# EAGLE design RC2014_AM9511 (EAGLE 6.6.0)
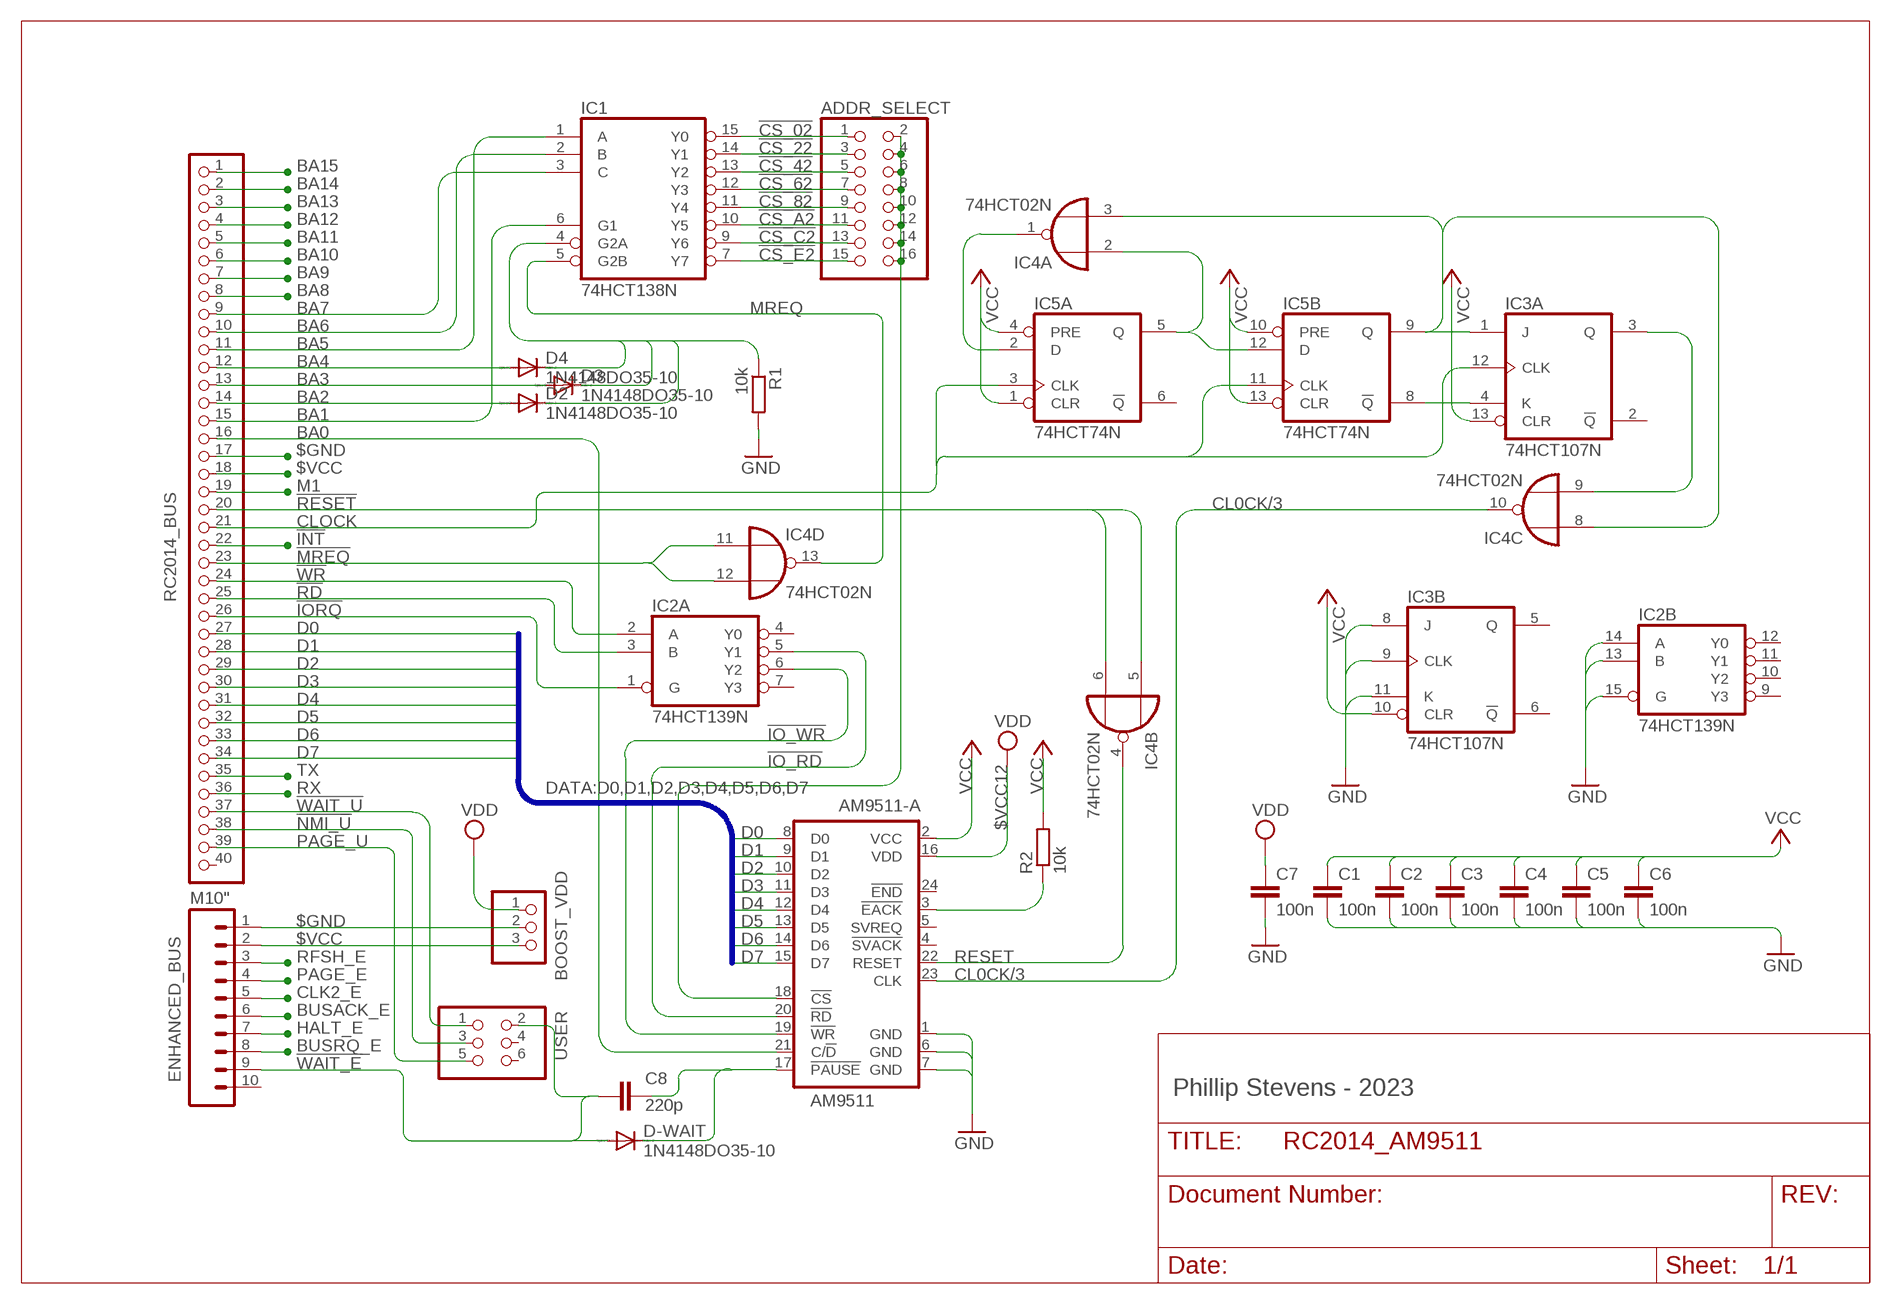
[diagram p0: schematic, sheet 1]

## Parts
ADDR_SELECT  PINHD-2X8  [2X08]
AM9511-A  AM9511  [DIL24-6]
BOOST_VDD  PINHD-1X3  [1X03]
C1  100n  C-EU025-025X050  [C025-025X050]
C2  100n  C-EU025-025X050  [C025-025X050]
C3  100n  C-EU025-025X050  [C025-025X050]
C4  100n  C-EU025-025X050  [C025-025X050]
C5  100n  C-EU025-025X050  [C025-025X050]
C6  100n  C-EU025-025X050  [C025-025X050]
C7  100n  C-EU025-025X050  [C025-025X050]
C8  220p  C-EU025-025X050  [C025-025X050]
D2  1N4148DO35-10  [DO35-10]
D3  1N4148DO35-10  [DO35-10]
D4  1N4148DO35-10  [DO35-10]
D-WAIT  1N4148DO35-10  [DO35-10]
ENHANCED_BUS  M10"  [1X10]
IC1  74HCT138N  [DIL16]
IC2  74HCT139N  [DIL16]
IC3  74HCT107N  [DIL14]
IC4  74HCT02N  [DIL14]
IC5  74HCT74N  [DIL14]
R1  10k  R-EU_0207/10  [0207/10]
R2  10k  R-EU_0207/10  [0207/10]
RC2014_BUS  RC2014 BUS  PINHD-1X40  [1X40]
USER  PINHD-2X3  [2X03]

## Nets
!CS: ADDR_SELECT.2 ADDR_SELECT.4 ADDR_SELECT.6 ADDR_SELECT.8 ADDR_SELECT.10 ADDR_SELECT.12 ADDR_SELECT.14 ADDR_SELECT.16 AM9511-A.18(!CS)
!CS_02: ADDR_SELECT.1 IC1.15(Y0)
!CS_22: ADDR_SELECT.3 IC1.14(Y1)
!CS_42: ADDR_SELECT.5 IC1.13(Y2)
!CS_62: ADDR_SELECT.7 IC1.12(Y3)
!CS_82: ADDR_SELECT.9 IC1.11(Y4)
!CS_A2: ADDR_SELECT.11 IC1.10(Y5)
!CS_C2: ADDR_SELECT.13 IC1.9(Y6)
!CS_E2: ADDR_SELECT.15 IC1.7(Y7)
!EACK: AM9511-A.3(!EACK) R2.1
!INT: RC2014_BUS.22
!IO_RD: AM9511-A.20(!RD) IC2.5(A:Y1)
!IO_WR: AM9511-A.19(!WR) IC2.6(A:Y2)
!IORQ: IC2.1(A:G) RC2014_BUS.26
!MREQ: IC4.11(D:I0) IC4.12(D:I1) RC2014_BUS.23
!NMI_U: RC2014_BUS.38 USER.3
!PAUSE: AM9511-A.17(!PAUSE) C8.1 D-WAIT.C
!RD: IC2.3(A:B) RC2014_BUS.25
!RESET: IC4.5(B:I0) IC4.6(B:I1) RC2014_BUS.20
!WAIT_E: C8.2 D-WAIT.A ENHANCED_BUS.9 USER.2
!WAIT_U: RC2014_BUS.37 USER.1
!WR: IC2.2(A:A) RC2014_BUS.24
$GND: AM9511-A.1(GND) AM9511-A.6(GND) AM9511-A.7(GND) BOOST_VDD.2 C1.2 C2.2 C3.2 C4.2 C5.2 C6.2 C7.2 ENHANCED_BUS.1 IC2.13(B:B) IC2.14(B:A) IC2.15(B:G) IC3.8(B:J) IC3.9(B:CLK) IC3.11(B:K) R1.2 RC2014_BUS.17 ; supply symbol labelled GND
$VCC: AM9511-A.2(VCC) BOOST_VDD.3 C1.1 C2.1 C3.1 C4.1 C5.1 C6.1 ENHANCED_BUS.2 IC3.10(B:CLR) IC3.13(A:CLR) IC5.1(A:CLR) IC5.4(A:PRE) IC5.10(B:PRE) IC5.13(B:CLR) R2.2 RC2014_BUS.18 ; supply symbol labelled VCC
$VCC12: AM9511-A.16(VDD) BOOST_VDD.1 C7.1 ; supply symbol labelled VDD
BA0: AM9511-A.21(C/!D) RC2014_BUS.16
BA1: IC1.6(G1) RC2014_BUS.15
BA2: D2.A RC2014_BUS.14
BA3: D3.A RC2014_BUS.13
BA4: D4.A RC2014_BUS.12
BA5: IC1.1(A) RC2014_BUS.11
BA6: IC1.2(B) RC2014_BUS.10
BA7: IC1.3(C) RC2014_BUS.9
BA8: RC2014_BUS.8
BA9: RC2014_BUS.7
BA10: RC2014_BUS.6
BA11: RC2014_BUS.5
BA12: RC2014_BUS.4
BA13: RC2014_BUS.3
BA14: RC2014_BUS.2
BA15: RC2014_BUS.1
BUSACK_E: ENHANCED_BUS.6
BUSRQ_E: ENHANCED_BUS.8
CL0CK/3: AM9511-A.23(CLK) IC4.10(C:O)
CLK2_E: ENHANCED_BUS.5
CLOCK: IC3.12(A:CLK) IC5.3(A:CLK) IC5.11(B:CLK) RC2014_BUS.21
D0: AM9511-A.8(D0) RC2014_BUS.27
D1: AM9511-A.9(D1) RC2014_BUS.28
D2: AM9511-A.10(D2) RC2014_BUS.29
D3: AM9511-A.11(D3) RC2014_BUS.30
D4: AM9511-A.12(D4) RC2014_BUS.31
D5: AM9511-A.13(D5) RC2014_BUS.32
D6: AM9511-A.14(D6) RC2014_BUS.33
D7: AM9511-A.15(D7) RC2014_BUS.34
HALT_E: ENHANCED_BUS.7
M1: RC2014_BUS.19
MREQ: IC1.5(G2B) IC4.13(D:O)
N$2: D2.C D3.C D4.C IC1.4(G2A) R1.1
N$3: IC4.2(A:I0) IC5.5(A:Q) IC5.12(B:D)
N$4: IC4.1(A:O) IC5.2(A:D)
N$5: IC3.3(A:Q) IC4.9(C:I1)
N$10: IC3.1(A:J) IC4.3(A:I1) IC4.8(C:I0) IC5.9(B:Q)
N$11: IC3.4(A:K) IC5.8(B:!Q)
PAGE_E: ENHANCED_BUS.4
PAGE_U: RC2014_BUS.39 USER.5
RESET: AM9511-A.22(RESET) IC4.4(B:O)
RFSH_E: ENHANCED_BUS.3
RX: RC2014_BUS.36
TX: RC2014_BUS.35
Unconnected: AM9511-A.4(!SVACK) AM9511-A.5(SVREQ) AM9511-A.24(!END) ENHANCED_BUS.10 IC2.4(A:Y0) IC2.7(A:Y3) IC2.9(B:Y3) IC2.10(B:Y2) IC2.11(B:Y1) IC2.12(B:Y0) IC3.2(A:!Q) IC3.5(B:Q) IC3.6(B:!Q) IC5.6(A:!Q) RC2014_BUS.40 USER.4 USER.6

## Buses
DATA:D0,D1,D2,D3,D4,D5,D6,D7

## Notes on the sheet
- Phillip Stevens - 2023

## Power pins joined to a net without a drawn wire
$GND: IC1.8(GND) IC2.8(P:GND) IC3.7(P:GND) IC4.7(P:GND) IC5.7(P:GND)
$VCC: IC1.16(VCC) IC2.16(P:VCC) IC3.14(P:VCC) IC4.14(P:VCC) IC5.14(P:VCC)

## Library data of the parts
ADDR_SELECT = pinhead:PINHD-2X8: PIN HEADER
AM9511-A = FX-Z180 Rev A:AM9511
BOOST_VDD = pinhead:PINHD-1X3: PIN HEADER
C1-C8 = rcl:C-EU: CAPACITOR, European symbol
D2-D4 D-WAIT = diode:1N4148: DIODE
ENHANCED_BUS = SparkFun:M10: Header 10 Standard 10-pin 0.1" header. Use with straight break away headers (SKU : PRT-00116), right angle break away headers (PRT-00553), swiss pins (PRT-00743), machine pins (PRT-00117), and female headers (PRT-00115).
IC1 = 74xx-eu:74*138: 3-line to 8-line DECODER/DEMULTIPLEXER
IC2 = 74xx-eu:74*139: Dual 2-line to 4-line DECODER/DEMULTIPLEXER
IC3 = 74xx-eu:74*107: Dual J-K FLIP FLOP, clear
IC4 = 74xx-eu:74*02: Quad 2-input NOR gate
IC5 = 74xx-eu:74*74: Dual D type positive edge triggered FLIP FLOP, preset and clear
R1 R2 = rcl:R-EU_: RESISTOR, European symbol
RC2014_BUS = pinhead:PINHD-1X40: PIN HEADER
USER = pinhead:PINHD-2X3: PIN HEADER

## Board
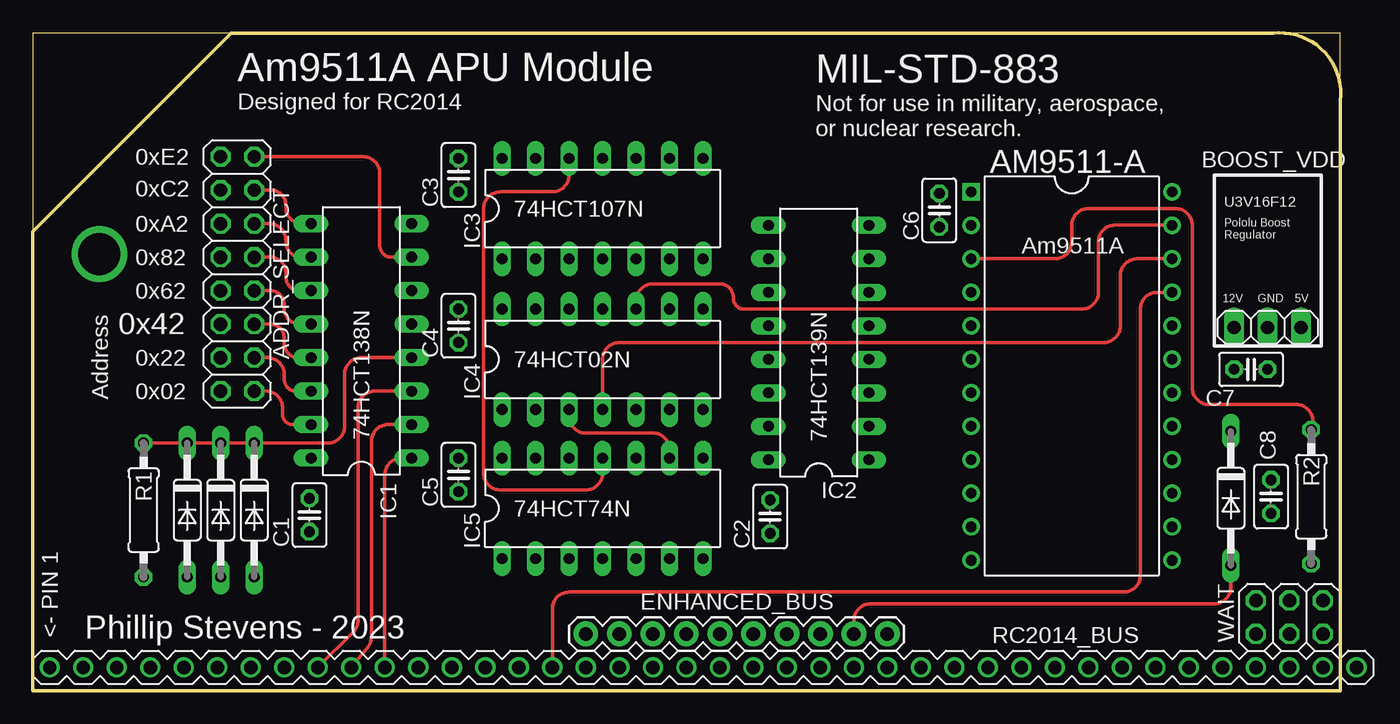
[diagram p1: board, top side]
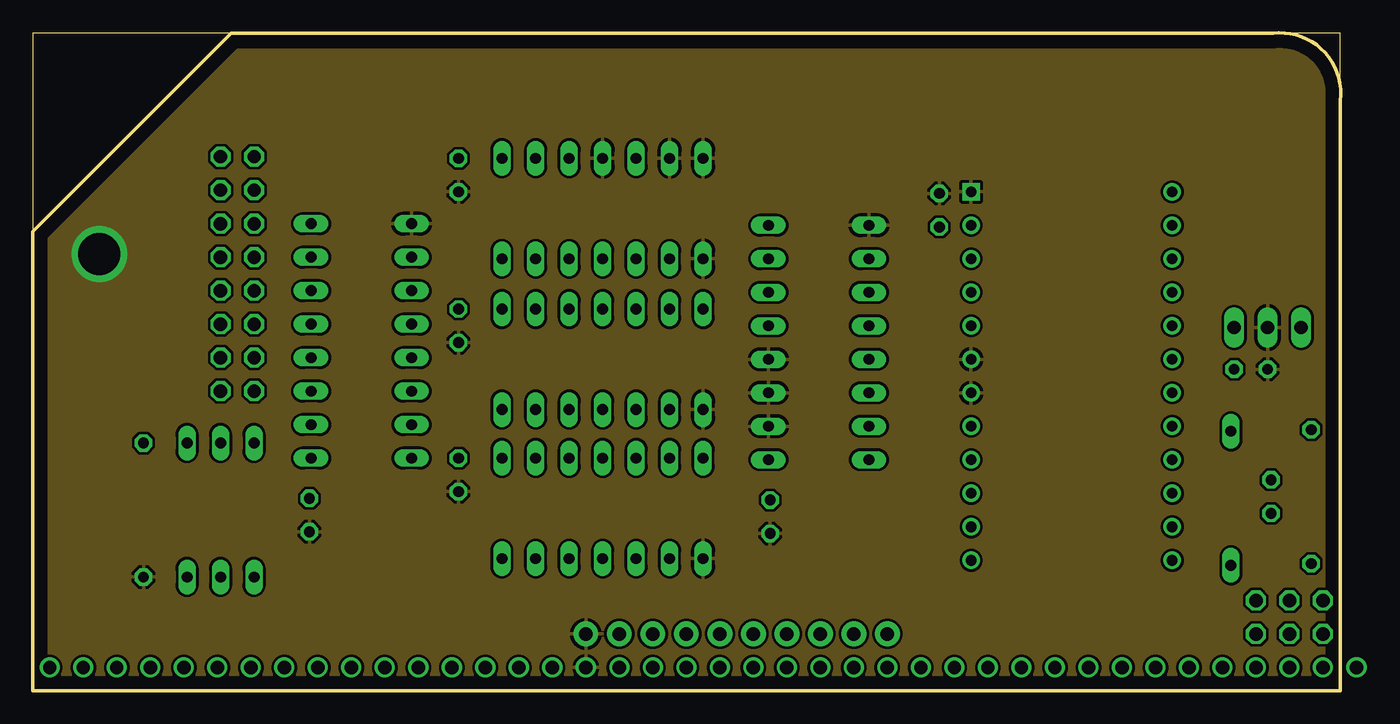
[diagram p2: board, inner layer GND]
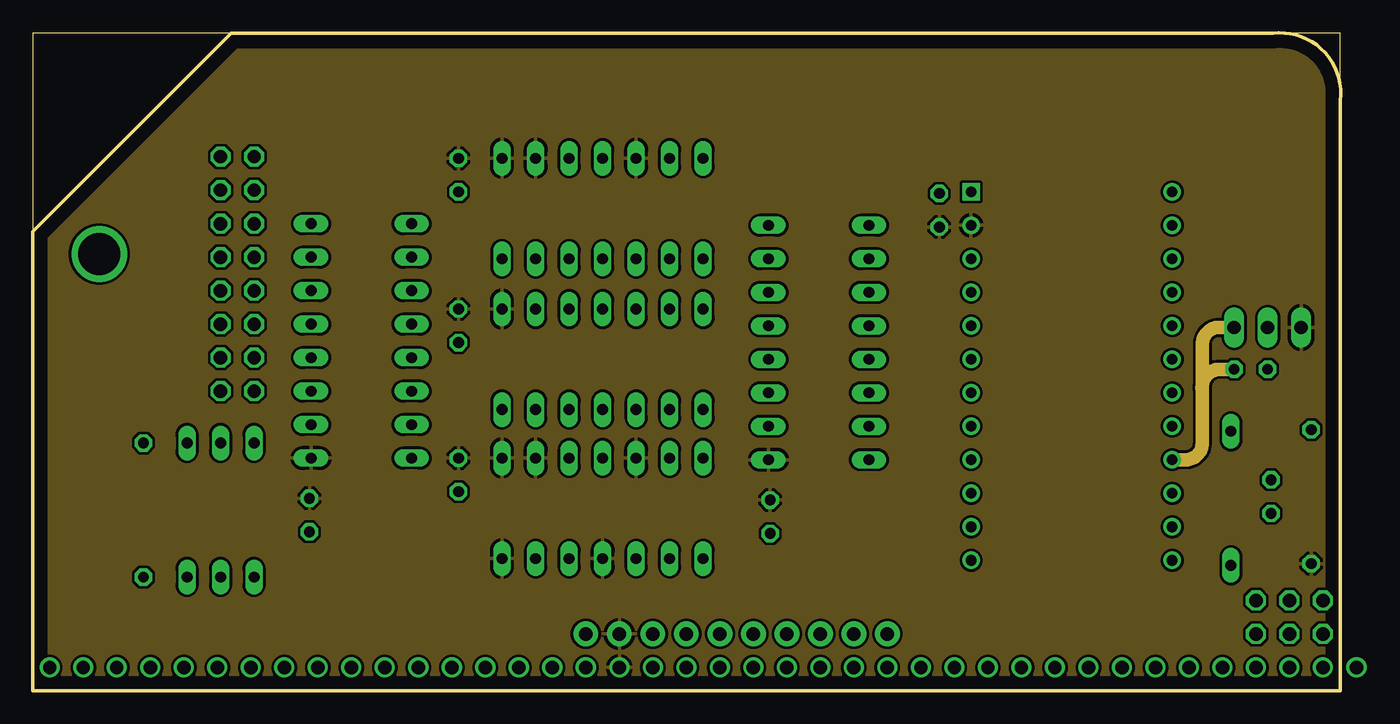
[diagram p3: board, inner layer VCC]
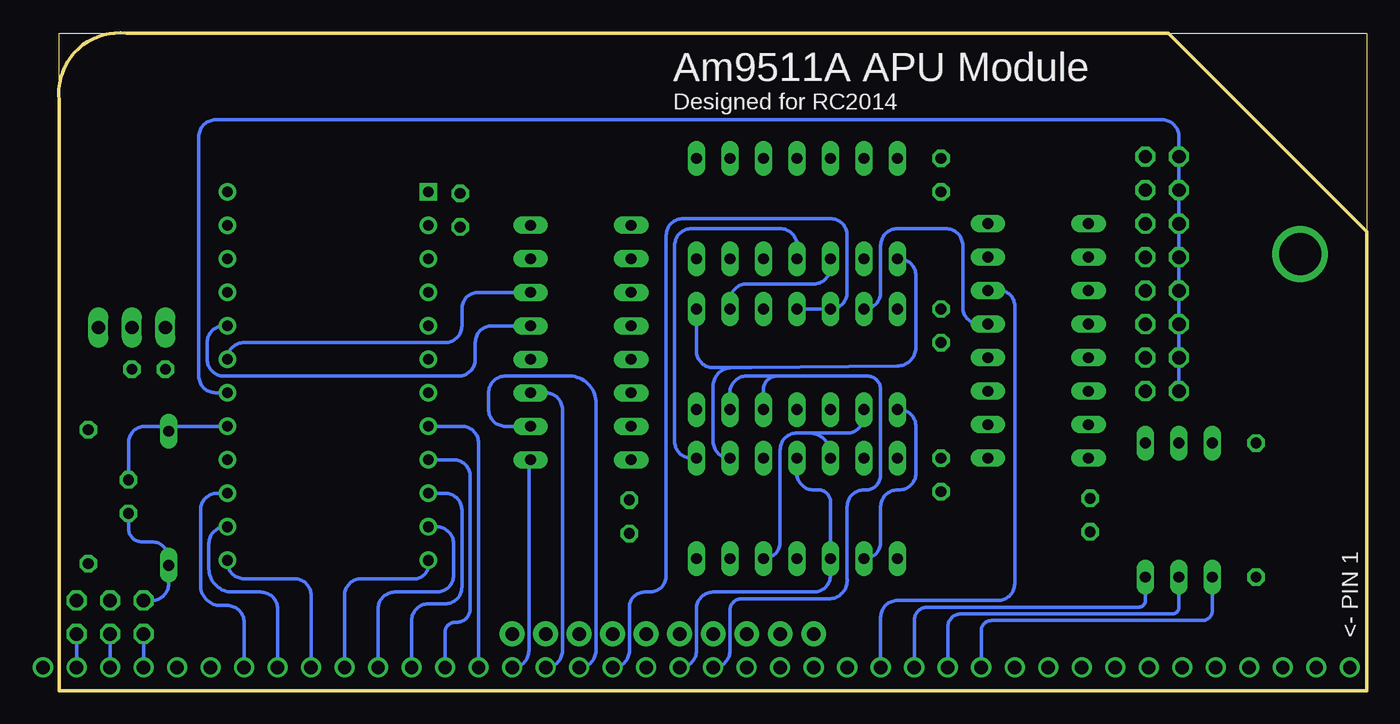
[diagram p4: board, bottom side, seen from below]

Size 99.14 x 49.89 mm. Coordinates in mm from the lower left corner, seen from the top.
Outline: 99.11,44.76 99.11,49.86 94.01,49.86
Outline: 15.01,49.86 0,49.86 0,34.85
Outline: 0,34.85 15.01,49.86
Outline: 94.01,49.86 arc-104 99.11,44.76
Outline: 15.01,49.86 94.01,49.86
Outline: 99.11,44.76 99.11,0 0,0 0,34.85
Copper layers (1*2*15*16): Top 0.035mm / dielectric 0.3mm / GND 0.035mm / dielectric 0.3mm / VCC 0.035mm / dielectric 0.3mm / Bottom 0.035mm
Design rules "default *": minimum track width 10mil, minimum drill 24mil, track to track 8mil, track to pad 8mil, pad to pad 8mil, via to via 8mil, smd to smd 8mil, copper to edge 40mil, drill to drill 8mil, minimum pad ring 10mil, minimum via ring 8mil, stop-mask expansion 4mil, vias tented up to drill 0mil, thermal gap 10mil

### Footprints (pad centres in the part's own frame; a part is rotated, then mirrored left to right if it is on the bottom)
2X08 = drill 1.016 octagon: 1 -8.89,-1.27; 2 -8.89,1.27; 3 -6.35,-1.27; 4 -6.35,1.27; 5 -3.81,-1.27; 6 -3.81,1.27; 7 -1.27,-1.27; 8 -1.27,1.27; 9 1.27,-1.27; 10 1.27,1.27; 11 3.81,-1.27; 12 3.81,1.27; 13 6.35,-1.27; 14 6.35,1.27; 15 8.89,-1.27; 16 8.89,1.27
DIL24-6 = drill 0.813 square: 1 -13.97,-7.62 | drill 0.813: 2 -11.43,-7.62; 3 -8.89,-7.62; 4 -6.35,-7.62; 5 -3.81,-7.62; 6 -1.27,-7.62; 7 1.27,-7.62; 8 3.81,-7.62; 9 6.35,-7.62; 10 8.89,-7.62; 11 11.43,-7.62; 12 13.97,-7.62; 13 13.97,7.62; 14 11.43,7.62; 15 8.89,7.62; 16 6.35,7.62; 17 3.81,7.62; 18 1.27,7.62; 19 -1.27,7.62; 20 -3.81,7.62; 21 -6.35,7.62; 22 -8.89,7.62; 23 -11.43,7.62; 24 -13.97,7.62
1X03 = drill 1.016 long: 1 -2.54,0; 2 0,0; 3 2.54,0
C025-025X050 = drill 0.813 octagon: 1 -1.27,0; 2 1.27,0
DO35-10 = drill 0.813 long: A 5.08,0; C -5.08,0
1X10 = drill 1.016 pad 1.88: 1 0,0; 2 2.54,0; 3 5.08,0; 4 7.62,0; 5 10.16,0; 6 12.7,0; 7 15.24,0; 8 17.78,0; 9 20.32,0; 10 22.86,0
DIL16 = drill 0.813 long: 1 -8.89,-3.81; 2 -6.35,-3.81; 3 -3.81,-3.81; 4 -1.27,-3.81; 5 1.27,-3.81; 6 3.81,-3.81; 7 6.35,-3.81; 8 8.89,-3.81; 9 8.89,3.81; 10 6.35,3.81; 11 3.81,3.81; 12 1.27,3.81; 13 -1.27,3.81; 14 -3.81,3.81; 15 -6.35,3.81; 16 -8.89,3.81
DIL14 = drill 0.813 long: 1 -7.62,-3.81; 2 -5.08,-3.81; 3 -2.54,-3.81; 4 0,-3.81; 5 2.54,-3.81; 6 5.08,-3.81; 7 7.62,-3.81; 8 7.62,3.81; 9 5.08,3.81; 10 2.54,3.81; 11 0,3.81; 12 -2.54,3.81; 13 -5.08,3.81; 14 -7.62,3.81
0207/10 = drill 0.813 octagon: 1 -5.08,0; 2 5.08,0
1X40 = drill 1.016: 1 -49.53,0; 2 -46.99,0; 3 -44.45,0; 4 -41.91,0; 5 -39.37,0; 6 -36.83,0; 7 -34.29,0; 8 -31.75,0; 9 -29.21,0; 10 -26.67,0; 11 -24.13,0; 12 -21.59,0; 13 -19.05,0; 14 -16.51,0; 15 -13.97,0; 16 -11.43,0; 17 -8.89,0; 18 -6.35,0; 19 -3.81,0; 20 -1.27,0; 21 1.27,0; 22 3.81,0; 23 6.35,0; 24 8.89,0; 25 11.43,0; 26 13.97,0; 27 16.51,0; 28 19.05,0; 29 21.59,0; 30 24.13,0; 31 26.67,0; 32 29.21,0; 33 31.75,0; 34 34.29,0; 35 36.83,0; 36 39.37,0; 37 41.91,0; 38 44.45,0; 39 46.99,0; 40 49.53,0
2X03 = drill 1.016 octagon: 1 -2.54,-1.27; 2 -2.54,1.27; 3 0,-1.27; 4 0,1.27; 5 2.54,-1.27; 6 2.54,1.27

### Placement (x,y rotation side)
ADDR_SELECT  15.49,31.62 90 top
AM9511-A  78.74,23.88 270 top
BOOST_VDD  93.6,27.56 0 top
C1  20.95,13.34 270 top
C2  55.88,13.21 270 top
C3  32.26,39.12 270 top
C4  32.26,27.69 270 top
C5  32.26,16.38 270 top
C6  68.71,36.45 90 top
C7  92.33,24.38 0 top
C8  93.85,14.73 270 top
D2  16.76,13.72 270 top
D3  14.22,13.72 270 top
D4  11.68,13.72 270 top
D-WAIT  90.81,14.61 270 top
ENHANCED_BUS  41.91,4.32 0 top
IC1  24.89,26.54 90 top
IC2  59.56,26.42 90 top
IC3  43.18,36.58 0 top
IC4  43.18,25.15 0 top
IC5  43.18,13.84 0 top
R1  8.38,13.72 270 top
R2  96.9,14.73 270 top
RC2014_BUS  50.8,1.78 0 top
USER  95.25,5.59 0 top

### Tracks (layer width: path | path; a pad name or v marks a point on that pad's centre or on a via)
!CS
  Bottom 0.254: ADDR_SELECT.10 ADDR_SELECT.8 ADDR_SELECT.6 ADDR_SELECT.4 ADDR_SELECT.2 ADDR_SELECT.10 | ADDR_SELECT.10 ADDR_SELECT.12 ADDR_SELECT.14 ADDR_SELECT.16 14.22,42.04 arc-90 15.49,43.31 87.25,43.31 arc-90 88.52,42.04 88.52,23.88 arc-90 87.25,22.61 AM9511-A.18
!CS_02
  Top 0.254: IC1.15 19.68,20.19 arc-90 18.92,20.95 18.92,21.46 arc90 17.65,22.73 ADDR_SELECT.1
!CS_22
  Top 0.254: IC1.14 19.94,22.73 arc-90 19.05,23.62 19.05,24 arc90 17.78,25.27 ADDR_SELECT.3
!CS_42
  Top 0.254: IC1.13 20.07,25.27 arc-90 19.05,26.42 19.05,26.8 arc90 17.91,27.81 ADDR_SELECT.5
!CS_62
  Top 0.254: IC1.12 20.19,27.81 arc-90 19.05,29.08 19.05,29.34 arc90 17.91,30.35 ADDR_SELECT.7
!CS_82
  Top 0.254: IC1.11 20.19,30.35 arc-90 19.18,31.37 19.18,31.75 arc90 17.91,32.89 ADDR_SELECT.9
!CS_A2
  Top 0.254: IC1.10 20.32,32.89 arc-90 19.18,34.04 19.18,34.16 arc90 17.91,35.43 ADDR_SELECT.11
!CS_C2
  Top 0.254: IC1.9 20.32,35.43 arc-90 19.18,36.7 19.18,36.83 arc90 18.03,37.97 ADDR_SELECT.13
!CS_E2
  Top 0.254: IC1.7 27.18,32.89 arc-90 26.29,33.78 26.29,39.24 arc90 25.02,40.51 ADDR_SELECT.15
!EACK
  Top 0.254: AM9511-A.3 77.47,32.77 arc90 78.74,34.04 78.74,35.31 arc-90 80.01,36.58 86.61,36.58 arc-90 87.88,35.31 87.88,22.99 arc90 89.15,21.72 95.76,21.72 arc-90 97.03,20.45 R2.1
!IO_RD
  Bottom 0.254: AM9511-A.20 86.61,27.69 arc-90 87.88,26.42 87.88,25.15 arc-90 86.61,23.88 68.83,23.88 arc-90 67.56,25.15 67.56,25.78 67.56,26.42 arc90 66.29,27.69 IC2.5
!IO_WR
  Bottom 0.254: AM9511-A.19 arc90 85.09,26.42 69.85,26.42 arc-90 68.58,27.69 68.58,28.07 68.58,28.96 arc90 67.31,30.23 IC2.6
!IORQ
  Bottom 0.254: RC2014_BUS.26 arc-90 63.5,3.05 63.5,17.4 arc90 IC2.1
!MREQ
  Bottom 0.254: RC2014_BUS.23 arc-90 55.88,3.05 55.88,6.35 arc90 54.74,7.49 54.36,7.49 arc-90 53.09,8.76 53.09,34.54 arc90 51.82,35.81 40.64,35.81 arc90 39.37,34.54 39.37,30.23 arc90 IC4.12 IC4.11
!NMI_U
  Bottom 0.254: RC2014_BUS.38 USER.3
!PAUSE
  Bottom 0.254: D-WAIT.C arc90 90.42,20.07 AM9511-A.17 92.58,20.07 arc-90 93.85,18.8 C8.1
!RD
  Bottom 0.254: RC2014_BUS.25 arc-90 60.96,3.05 60.96,21.34 arc-90 62.23,22.61 IC2.3
!RESET
  Bottom 0.254: RC2014_BUS.20 arc-90 48.26,3.05 48.26,6.1 arc90 47.37,6.99 40.64,6.99 arc-90 39.37,8.51 39.37,13.97 arc90 38.1,15.24 37.97,15.24 arc-90 36.83,16.38 36.83,22.86 arc-90 37.85,23.88 44.7,23.88 | 44.7,23.88 arc-90 45.72,22.86 IC4.5 | IC4.6 48.26,22.61 arc90 46.99,23.88 44.7,23.88
!WAIT_E
  Top 0.254: ENHANCED_BUS.9 62.23,5.33 arc-90 63.5,6.6 89.53,6.6 arc90 90.81,7.87 D-WAIT.A
  Bottom 0.254: USER.2 92.08,6.86 arc-90 90.81,8.13 D-WAIT.A 90.81,10.03 arc-90 92.08,11.3 92.84,11.3 arc90 93.85,12.32 C8.2
!WAIT_U
  Bottom 0.254: RC2014_BUS.37 USER.1
!WR
  Bottom 0.254: RC2014_BUS.24 arc-90 58.42,3.05 58.42,21.97 arc-90 60.58,23.88 65.28,23.88 arc-90 66.55,22.61 66.55,21.34 arc-90 65.28,20.07 IC2.2
$GND  (via drill 3.2)
  other vias: 5.03,33.12
  pour GND: 14.61,49.53 95.25,49.53 arc-90 99.06,45.72 99.06,0 0,0 0,34.92
$VCC
  pour VCC: 14.99,49.91 94.61,49.91 arc-90 99.06,45.72 99.06,0 0,0 0,34.92
$VCC12
  VCC 1.016: BOOST_VDD.1 89.92,27.56 arc90 88.65,26.29 88.65,22.73 | AM9511-A.16 87.38,17.53 arc90 88.65,18.8 88.65,22.73 | C7.1 89.79,24.38 arc90 88.65,22.73
BA0
  Top 0.254: RC2014_BUS.16 39.37,6.22 arc-90 40.64,7.49 82.68,7.49 arc90 83.95,8.76 83.95,28.96 arc-90 85.22,30.23 AM9511-A.21
BA1
  Bottom 0.254: RC2014_BUS.15 36.83,5.59 arc90 35.56,6.86 27.94,6.86 arc-90 26.67,8.13 26.67,29.21 arc-90 27.81,30.35 IC1.6
BA2
  Bottom 0.254: RC2014_BUS.14 34.29,5.33 arc90 33.27,6.35 17.27,6.35 arc-90 16.76,6.86 D2.A
BA3
  Bottom 0.254: RC2014_BUS.13 31.75,4.83 arc90 30.73,5.84 14.73,5.84 arc-90 14.22,6.35 D3.A
BA4
  Bottom 0.254: RC2014_BUS.12 29.21,4.57 arc90 28.45,5.33 12.45,5.33 arc-90 11.68,6.1 D4.A
BA5
  Top 0.254: IC1.1 27.94,17.65 arc90 26.67,16.38 RC2014_BUS.11
BA6
  Top 0.254: IC1.2 26.92,20.19 arc90 25.65,18.92 25.65,4.08 arc-45 25.28,3.18 RC2014_BUS.10
BA7
  Top 0.254: IC1.3 25.91,22.73 arc90 24.64,21.46 24.64,5.35 arc-45 24.27,4.45 RC2014_BUS.9
CL0CK/3
  Top 0.254: AM9511-A.23 82.04,35.31 arc90 80.77,34.16 80.77,30.23 arc-90 79.5,28.96 53.98,28.96 arc-90 53.09,29.72 arc90 52.2,30.86 46.99,30.86 arc90 45.72,29.59 IC4.10
CLOCK
  Top 0.254: IC3.12 40.64,39.12 arc-90 39.37,37.85 35.43,37.85 arc90 34.16,36.58 34.16,16.51 arc90 35.43,15.24 41.91,15.24 arc90 43.18,16.51 IC5.11
  Bottom 0.254: IC5.11 43.18,16.51 arc-90 41.91,15.24 41.53,15.24 arc90 40.64,14.35 IC5.3 40.64,8.76 arc90 41.91,7.49 49.53,7.49 arc-90 50.8,6.22 50.8,3.05 arc90 RC2014_BUS.21
D0
  Bottom 0.254: RC2014_BUS.27 67.31,18.8 arc-90 68.58,20.07 AM9511-A.8
D1
  Bottom 0.254: RC2014_BUS.28 69.85,4.45 arc90 69.09,5.21 68.96,5.21 arc-90 67.94,6.22 | 67.94,6.1 67.94,6.22 | 67.94,6.22 67.94,16.26 arc-90 69.22,17.53 AM9511-A.9
D2
  Bottom 0.254: RC2014_BUS.29 72.39,5.33 arc90 71.12,6.6 69.85,6.6 arc-90 68.58,7.87 68.58,13.72 arc-90 69.85,14.99 AM9511-A.10
D3
  Bottom 0.254: RC2014_BUS.30 74.93,6.22 arc90 73.66,7.49 70.48,7.49 arc-90 69.22,8.76 69.22,11.18 arc-90 70.48,12.45 AM9511-A.11
D4
  Bottom 0.254: RC2014_BUS.31 77.47,7.24 arc90 76.2,8.51 72.01,8.51 arc-90 71.12,9.78 AM9511-A.12
D5
  Bottom 0.254: RC2014_BUS.32 80.01,7.24 arc-90 81.28,8.51 85.09,8.51 arc90 86.36,9.78 AM9511-A.13
D6
  Bottom 0.254: RC2014_BUS.33 82.55,6.22 arc-90 83.82,7.49 85.98,7.49 arc90 87.76,9.27 87.76,11.18 arc90 86.49,12.45 AM9511-A.14
D7
  Bottom 0.254: RC2014_BUS.34 85.09,5.21 arc-90 86.36,6.48 86.87,6.48 arc90 88.39,8 88.39,13.72 arc90 87.12,14.99 AM9511-A.15
MREQ
  Bottom 0.254: IC1.5 29.34,27.81 arc90 30.61,29.08 30.61,33.78 arc-90 31.88,35.05 35.56,35.05 arc-90 36.83,33.78 36.83,30.23 arc90 IC4.13
N$2
  Top 0.254: IC1.4 24.89,25.27 arc90 23.62,24 23.62,20.07 arc-90 22.35,18.8 D2.C D3.C D4.C R1.1
N$3
  Bottom 0.254: IC5.5 arc-90 44.45,11.3 44.45,18.29 arc90 43.18,19.56 43.05,19.56 42.29,19.56 | 42.29,19.56 arc98 IC5.12 | IC4.2 38.1,20.83 arc90 39.37,19.56 42.29,19.56
N$4
  Bottom 0.254: IC5.2 arc-90 36.83,11.3 36.83,13.97 arc90 35.56,15.24 35.43,15.24 arc-90 34.16,16.51 34.16,20.07 arc-90 35.43,21.34 IC4.1
N$5
  Bottom 0.254: IC4.9 48.26,29.59 arc90 46.99,30.86 41.91,30.86 arc-90 40.64,32.13 IC3.3
N$10
  Top 0.254: IC4.3 40.64,20.83 arc90 41.91,19.56 46.99,19.56 arc-90 48.26,18.29 IC5.9
  Bottom 0.254: 49.53,24.51 arc90 50.8,25.78 | 50.8,25.78 arc-90 49.53,24.51 | 49.53,24.51 48.13,24.51 | 50.8,25.78 IC4.8 | IC5.9 arc90 49.53,18.92 49.53,23.11 arc90 48.13,24.51 | 48.13,24.51 46.61,24.51 35.56,24.64 arc-90 34.16,26.04 34.16,31.5 arc-90 35.43,32.77 IC3.1
N$11
  Bottom 0.254: IC5.8 51.18,17.65 arc90 52.45,18.92 52.45,33.78 arc90 51.18,35.05 44.45,35.05 arc90 43.18,33.78 IC3.4
PAGE_U
  Bottom 0.254: RC2014_BUS.39 USER.5
RESET
  Top 0.254: AM9511-A.22 83.69,32.77 arc90 82.42,31.5 82.42,27.69 arc-90 81.15,26.42 66.15,26.42 65.79,26.42 44.45,26.42 arc90 43.18,25.15 IC4.4

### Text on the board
tPlace: Am9511A APU Module | MIL-STD-883 | Designed for RC2014 | Not for use in military, aerospace, / or nuclear research. | 0xE2 | 0xC2 | U3V16F12 | 74HCT107N | 0xA2 | Pololu Boost / Regulator | Am9511A | 0x82 | 0x62 | 12V | GND | 5V | 0x42 | 0x22 | 74HCT02N | Address | 0x02 | 74HCT138N | 74HCT139N | 74HCT74N | <- PIN 1 | Phillip Stevens - 2023 | WAIT
bPlace: Am9511A APU Module | Designed for RC2014 | <- PIN 1

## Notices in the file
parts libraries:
SparkFun: Licensing: CC v3.0 Share-Alike You are welcome to use this library for commercial purposes.
